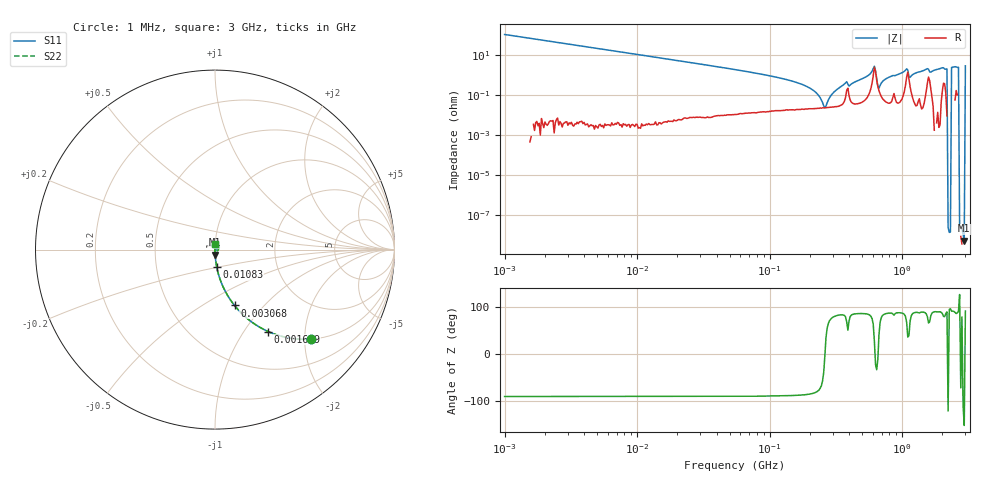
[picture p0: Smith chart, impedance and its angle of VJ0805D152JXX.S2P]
! VJ0805D152JXX
! DATE
! CORRECTED  DATA
# Hz  S  MA  R  50
!Freq	S11M	S11A	S21M	S21A	S12M	S12A	S22M	S22A
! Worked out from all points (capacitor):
!   401 points, 1 MHz to 3 GHz, reference 50 ohm
!   read as one part in series: C = 1.49 nF near 1.041 MHz
!   lowest |Z| = 5.06 nohm at 2.941 GHz (marker M1)
!   series resonance near 261.4 MHz, so ESL is about 250 pH
!   S11 on the Smith chart (normalised r, x): 1 MHz: 1.00, -2.14; 1.649 MHz: 1.00, -1.30; 3.068 MHz: 1.00, -0.70; 10.83 MHz: 1.00, -0.20; 3 GHz: 1.00, +0.06
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1000000  0.7311 -43.0  0.6824 47.0  0.6824 47.0  0.7311 -43.0
1649378  0.5447 -57.0  0.8386 33.0  0.8386 33.0  0.5447 -57.0
3067588  0.3297 -70.7  0.9441 19.2  0.9441 19.2  0.3297 -70.7
3823119  0.2698 -74.3  0.9629 15.7  0.9629 15.7  0.2698 -74.3
1.082539e7  0.09828 -84.3  0.9951 5.6  0.9951 5.6  0.09828 -84.3
1.461624e7  0.07283 -85.8  0.9973 4.2  0.9973 4.2  0.07283 -85.8
5.587962e7  0.01825 -88.6  0.9997 1.0  0.9997 1.0  0.01825 -88.6
1.375402e8  0.005639 -87.9  0.9998 0.3  0.9998 0.3  0.005639 -87.9
2.094008e8  0.001864 -83.6  0.9998 0.1  0.9998 0.1  0.001864 -83.6
2.609752e8  0.0002274 -3.8  0.9998 0.0  0.9998 0.0  0.0002274 -3.8
3.002264e8  0.001233 78.3  0.9998 -0.1  0.9998 -0.1  0.001233 78.3
3.667557e8  0.003538 81.9  0.9995 -0.2  0.9995 -0.2  0.003538 81.9
4.135554e8  0.003539 82.8  0.9996 -0.2  0.9996 -0.2  0.003539 82.8
6.049187e8  0.02056 62.2  0.9906 -1.1  0.9906 -1.1  0.02056 62.2
6.821091e8  0.003027 68.3  0.9989 -0.2  0.9989 -0.2  0.003027 68.3
8.005644e8  0.007858 86.7  0.9996 -0.4  0.9996 -0.4  0.007858 86.7
1.059487e9  0.01734 79.0  0.9968 -1.0  0.9968 -1.0  0.01734 79.0
1.171007e9  0.008972 80.9  0.9986 -0.5  0.9986 -0.5  0.008972 80.9
1.519029e9  0.01936 84.4  0.9983 -1.1  0.9983 -1.1  0.01936 84.4
1.67892e9  0.01522 86.2  0.9991 -0.9  0.9991 -0.9  0.01522 86.2
2.940549e9  0.02846 -88.6  1.001 -1.6  1.001 -1.6  0.02846 -88.6
3e9  0.02873 89.9  1 -1.6  1 -1.6  0.02873 89.9
